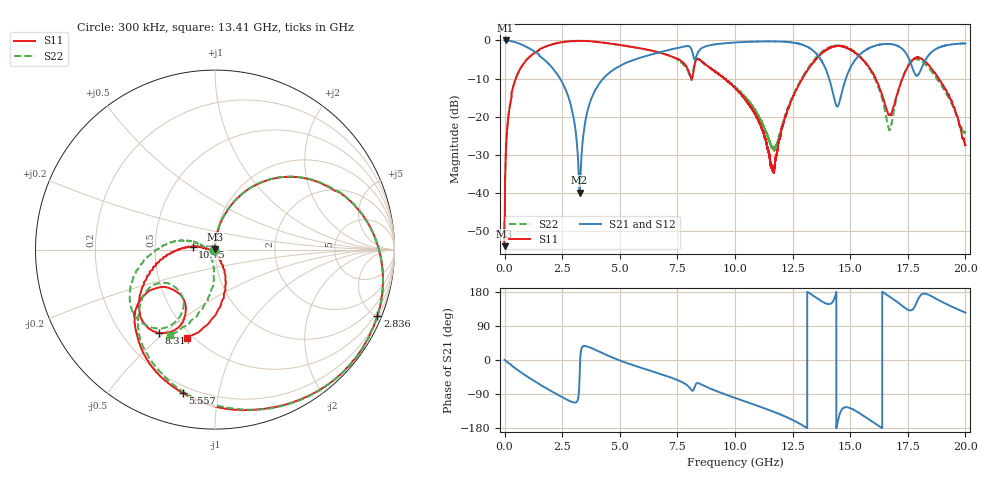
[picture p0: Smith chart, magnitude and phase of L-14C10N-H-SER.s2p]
!{L-14C10N}
!Johanson Technology Inc.
!www.johansontechnology.com
!Test Board Conditions:
!Substrate Type  RO4350B
!Substrate Thickness  20 mil
!Substrate Dk  3.66
!TL Type: GCPW
!TL Trace Width  36 mil
!TL Gap  12 mil
!Electrode orientation  Horizontal
!DUT TOPOLOGY	SERIES
!Mounting Pad LxW  26x36 mil
! Created Sun Jun 20 13:00:22 2021
# hz S ma R 50
! 2 Port Network Data from SP1.SP block
! freq  magS11  angS11  magS21  angS21  magS12  angS12  magS22  angS22
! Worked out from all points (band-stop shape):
!   20001 points, 300 kHz to 20 GHz, reference 50 ohm
!   highest |S21| = 0.00 dB at 39.3 MHz (marker M1); lowest = -39.8 dB at 3.256 GHz (marker M2)
!   |S21| within 3 dB of the highest: 8.404 GHz to 13.45 GHz (5.049 GHz wide, 46.2 % of centre); 15.55 GHz to 17.38 GHz (1.829 GHz wide, 11.1 % of centre)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
!   lowest |S11| = -53.9 dB at 1.3 MHz (marker M3), VSWR 1.00, Z = 49.8 + j0.11 ohm
!   |S11| at or under -10 dB: 9.543 GHz to 12.92 GHz (3.375 GHz wide, 30 % of centre); 16.11 GHz to 17.27 GHz (1.161 GHz wide, 6.96 % of centre); 18.84 GHz to end of sweep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
!   |S22| runs from -53.0 to -0.1 dB; largest |S21 - S12| = 0.013
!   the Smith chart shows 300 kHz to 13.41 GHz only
!   S11 on the Smith chart (normalised r, x): 300 kHz: 0.99, -0.00; 2.836 GHz: 0.32, -5.11; 5.557 GHz: 0.16, -0.79; 8.317 GHz: 0.36, -0.48; 10.75 GHz: 0.78, +0.03; 13.41 GHz: 0.46, -0.63
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300000  0.004169 -161.4  0.9968 0.2  0.9954 0.2  0.004107 -154.1
1300000  0.002023 146.8  0.9983 0.0  0.9983 0.0  0.002241 141.8
3.93e7  0.02547 88.2  0.9997 -1.8  0.9991 -1.9  0.02568 88.3
2.153e8  0.1321 79.7  0.9894 -9.7  0.989 -9.7  0.133 79.7
6.073e8  0.3872 60.9  0.9161 -28.1  0.9153 -28.2  0.3878 61.0
2.8363e9  0.9767 -22.1  0.1567 -108.5  0.1573 -108.6  0.9774 -21.9
3.2563e9  0.9885 -37.4  0.01019 -40.2  0.01033 -39.6  0.9894 -37.3
3.3343e9  0.9884 -40.1  0.02946 29.1  0.02956 29.3  0.9892 -40.0
3.9103e9  0.9626 -59.4  0.2169 27.6  0.2166 27.6  0.9665 -59.2
5.5573e9  0.8177 -102.7  0.5503 -13.3  0.5498 -13.4  0.8219 -100.7
6.6673e9  0.7035 -124.5  0.6914 -35.2  0.693 -35.0  0.6985 -122.4
8.3173e9  0.5577 -123.8  0.6144 -62.5  0.6161 -62.2  0.5745 -133.8
1.00003e10  0.2401 -176.1  0.9383 -100.0  0.9396 -100.1  0.2477 170.6
1.07453e10  0.1257 172.1  0.9612 -115.9  0.9632 -116.0  0.1408 160.5
1.16433e10  0.02117 -124.9  0.9699 -135.9  0.9696 -135.9  0.03951 -157.5
1.33343e10  0.4878 -104.1  0.7592 172.2  0.7631 171.9  0.5085 -115.1
1.34073e10  0.522 -107.5  0.7275 169.3  0.7317 168.8  0.543 -118.2
1.44423e10  0.8466 -170.6  0.1369 -167.8  0.1372 -168.4  0.8535 -169.3
1.54523e10  0.5997 138.0  0.6677 -142.5  0.6588 -142.6  0.6032 141.9
1.66673e10  0.1063 153.4  0.9012 168.9  0.8993 169.2  0.0712 146.8
1.78953e10  0.5989 161.6  0.3448 153.4  0.3472 154.4  0.5691 141.4
2e10  0.04298 142.2  0.914 125.1  0.9097 125.0  0.06238 122.0
